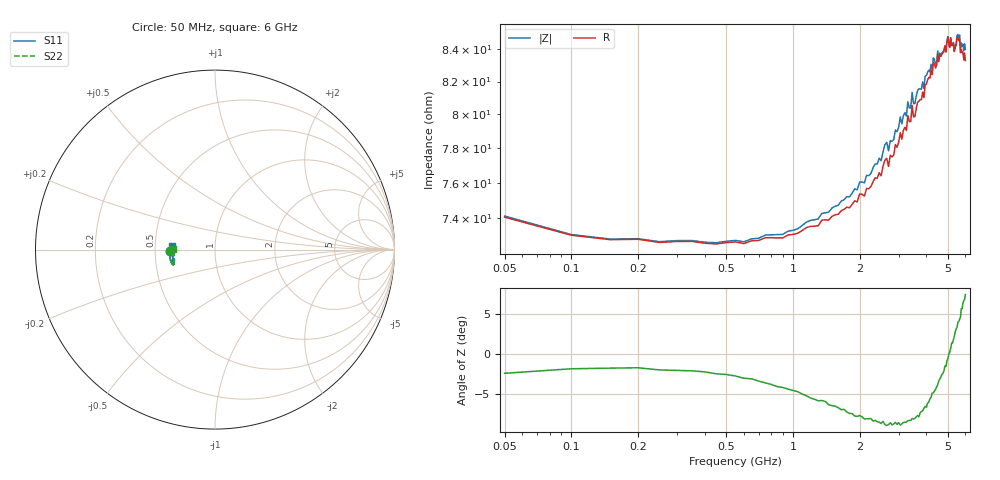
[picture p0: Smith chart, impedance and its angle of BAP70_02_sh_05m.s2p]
!	Created	by	janssen	on	Thu	Dec	12	13:21:33	MET	2002
#	HZ	S	MA	R	50
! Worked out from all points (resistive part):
!   120 points, 50 MHz to 6 GHz, reference 50 ohm
!   read as one part in shunt: R = 74.1 ohm at 50 MHz
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5e7  0.2527 -178.2  0.7489 -0.5  0.7473 -0.7  0.2531 -178.1
1.05e9  0.2556 -170.8  0.7451 0.6  0.7445 0.5  0.2547 -170.5
2.05e9  0.2531 -164.6  0.7524 1.1  0.7496 1.0  0.2535 -163.2
2.7e9  0.2536 -162.4  0.7568 1.4  0.7536 1.3  0.2488 -160.6
3e9  0.2503 -161.8  0.7602 1.6  0.7579 1.5  0.2476 -160.5
3.05e9  0.2448 -162.1  0.7597 1.3  0.7555 1.4  0.2443 -160.1
3.1e9  0.249 -161.4  0.7602 1.6  0.7569 1.4  0.2469 -160.1
3.3e9  0.2465 -162.0  0.7629 1.6  0.7598 1.6  0.2421 -160.2
3.35e9  0.2451 -161.8  0.7631 1.7  0.7585 1.6  0.2465 -160.5
3.45e9  0.2468 -162.0  0.7652 1.8  0.7605 1.6  0.2405 -160.3
3.5e9  0.2471 -162.0  0.7642 1.7  0.7594 1.6  0.2442 -160.5
3.6e9  0.2495 -162.4  0.7663 1.8  0.7608 1.6  0.2415 -160.6
3.8e9  0.2447 -163.2  0.7666 1.8  0.7631 1.8  0.2429 -161.4
4.05e9  0.2431 -165.0  0.7691 1.9  0.7644 1.9  0.2374 -162.2
5e9  0.2356 -172.8  0.7771 2.1  0.7714 2.3  0.2311 -169.6
5.05e9  0.239 -173.5  0.7764 2.2  0.7706 2.2  0.229 -170.2
5.65e9  0.2358 179.5  0.7799 2.1  0.7742 2.4  0.2302 -176.9
5.7e9  0.2434 179.6  0.7796 2.2  0.775 2.4  0.2298 -177.6
5.8e9  0.2382 177.8  0.7794 2.2  0.7741 2.4  0.232 -179.0
5.85e9  0.241 176.3  0.78 2.3  0.7737 2.5  0.2285 -179.5
5.9e9  0.2407 176.1  0.7799 2.2  0.7752 2.5  0.2333 179.8
6e9  0.2418 175.0  0.781 2.3  0.7761 2.5  0.2332 179.2
